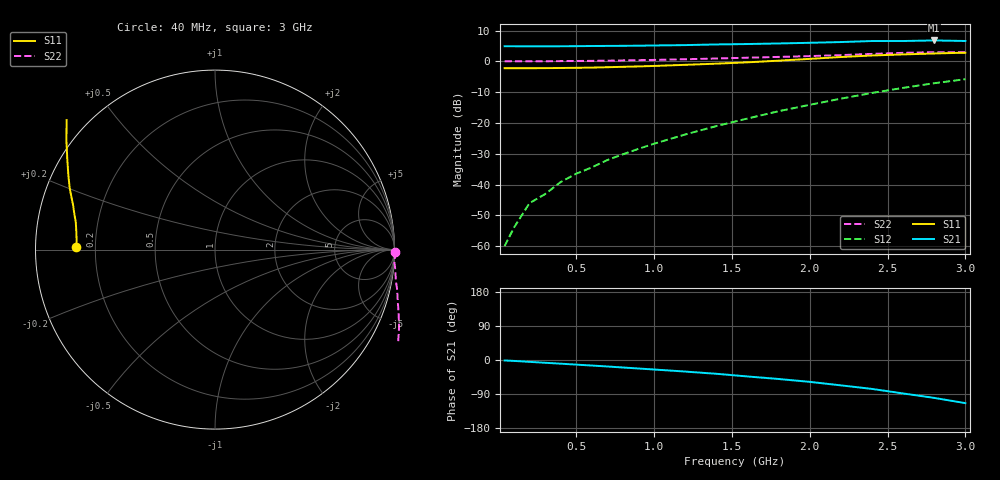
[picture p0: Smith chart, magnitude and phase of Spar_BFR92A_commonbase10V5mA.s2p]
! Filename:  BFR92ACG.S2P  Version:  2.0
! NXP part #: BFR92A  Date: Jul 1990
! Bias condition: Vce=10V, Ic=5mA
! COMMON BASE
#  MHz  S  MA  R  50
! Freq  S11  S21  S12  S22
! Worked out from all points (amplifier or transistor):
!   21 points, 40 MHz to 3 GHz, reference 50 ohm
!   highest |S21| = 6.8 dB at 2.8 GHz (marker M1)
!   |S21| within 3 dB of that: start of sweep to end of sweep
!   unconditionally stable (mu >= 1): nowhere
!   at 300 MHz: K = -0.40, MSG = 24.0 dB, |S12| = -43.1 dB
!   at 1 GHz: K = -0.90, MSG = 15.9 dB, |S12| = -26.7 dB
!   at 3 GHz: K = -0.77, MSG = 6.2 dB, |S12| = -5.8 dB
40  0.774 178.9  1.76 -1.2  0.001 61.3  1.002 -0.7
100  0.772 177.9  1.758 -2.4  0.002 86.3  1.004 -1.3
200  0.773 176.0  1.755 -4.9  0.005 103.5  1.003 -3.0
300  0.776 174.1  1.754 -7.3  0.007 110.5  1.003 -4.4
400  0.78 172.3  1.758 -9.7  0.011 119.0  1.009 -5.9
500  0.785 170.5  1.763 -12.2  0.015 122.6  1.014 -7.4
600  0.792 168.5  1.774 -14.6  0.019 127.7  1.019 -8.9
700  0.803 166.7  1.78 -17.1  0.025 131.0  1.026 -10.4
800  0.815 164.7  1.786 -19.8  0.031 133.7  1.036 -11.9
900  0.827 162.8  1.794 -22.4  0.038 135.7  1.046 -13.7
1000  0.842 161.0  1.81 -25.1  0.046 138.0  1.055 -15.3
1200  0.878 157.2  1.835 -30.5  0.065 140.0  1.081 -18.9
1400  0.917 153.0  1.881 -36.4  0.089 140.2  1.112 -22.7
1600  0.964 148.6  1.91 -43.4  0.118 140.0  1.145 -27.0
1800  1.026 143.8  1.951 -50.1  0.155 138.3  1.181 -31.9
2000  1.097 138.9  2 -57.7  0.197 135.8  1.217 -37.8
2200  1.175 133.6  2.057 -66.9  0.248 132.6  1.263 -44.7
2400  1.245 127.8  2.137 -76.3  0.307 128.1  1.32 -52.5
2600  1.296 120.5  2.139 -88.3  0.371 123.2  1.374 -60.7
2800  1.342 111.5  2.183 -100.0  0.442 116.5  1.411 -69.2
3000  1.382 101.9  2.14 -113.8  0.513 109.8  1.41 -78.7
